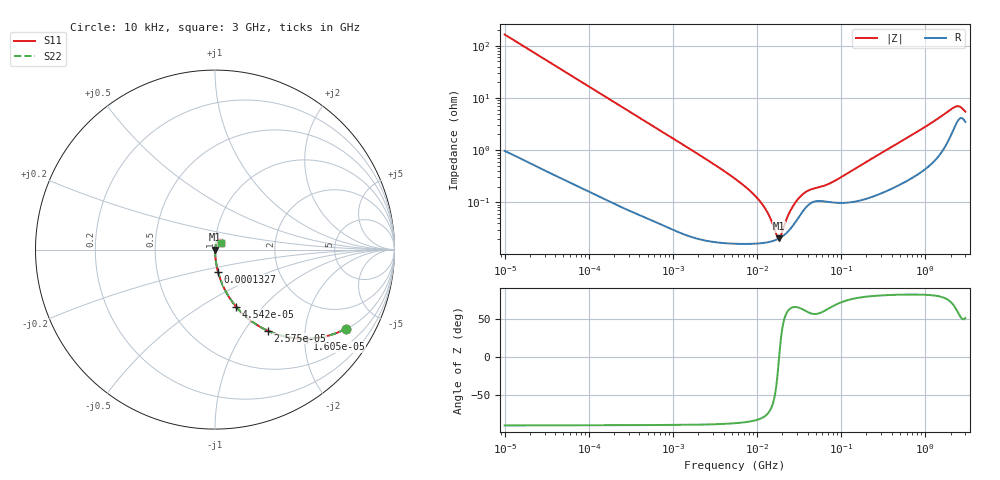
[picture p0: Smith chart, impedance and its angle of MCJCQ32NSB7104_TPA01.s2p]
! MCJCQ32NSB7104_TPA01  S-PARAMETER MODEL  ( Standard Model )
! Model Generated by TAIYO YUDEN Corporation (http://www.ty-top.com)
! Version 1.0
! TAIYO YUDEN Control No. 220601
! Copyright(c) 2015 TAIYO YUDEN CO.,LTD. All Rights Reserved.
! Product Description (link to TY-COMPAS)
! https://ds.yuden.co.jp/TYCOMPAS/or/detail?pn=MCJCQ32NSB7104KTPA01&u=M
! Products Name : Multilayer Ceramic Capacitors
! Characteristics :
!  Capacitance : 0.1 [uF] , Rated Voltage : 250 [V] , TCC : X7R
!  Case Size : 3.2 x 2.5 / 0.126 x 0.098 [mm/inch] , Thickness : 1.9 / 0.075 [mm/inch]
!  (Conditions: Temperature = 25 [degC] , DC Bias Voltage = 0 [V])
! External Node Assignments :
!  1  o---| |---o  2
! GND o---------o GND
! Frequency Range : 10kHz  -  3GHz  [ 401 STEP ]
# MHZ S RI R 50
! Freq[MHz].  S11 Real  S11 Imag  S21 Real  S21 Imag  S12 Real  S12 Imag  S22 Real  S22 Imag
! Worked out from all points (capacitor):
!   401 points, 10 kHz to 3 GHz, reference 50 ohm
!   read as one part in series: C = 96.7 nF near 10.65 kHz
!   lowest |Z| = 20.4 mohm at 18.15 MHz (marker M1)
!   series resonance near 18.34 MHz, so ESL is about 780 pH
!   S11 on the Smith chart (normalised r, x): 10 kHz: 1.02, -3.29; 16.05 kHz: 1.01, -2.05; 25.75 kHz: 1.01, -1.28; 45.42 kHz: 1.01, -0.73; 132.7 kHz: 1.00, -0.25; 3 GHz: 1.07, +0.08
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0.01  0.7287 -0.4417  0.2713 0.4417  0.2713 0.4417  0.7287 -0.4417
0.016047  0.513 -0.4966  0.487 0.4966  0.487 0.4966  0.513 -0.4966
0.02575  0.2925 -0.4514  0.7075 0.4514  0.7075 0.4514  0.2925 -0.4514
0.045421  0.1192 -0.3199  0.8808 0.3199  0.8808 0.3199  0.1192 -0.3199
0.082683  0.0404 -0.1923  0.9596 0.1923  0.9596 0.1923  0.0404 -0.1923
0.132681  0.0167 -0.1232  0.9833 0.1232  0.9833 0.1232  0.0167 -0.1232
0.683653  0.000997 -0.0246  0.999 0.0246  0.999 0.0246  0.000997 -0.0246
5.477226  0.000169 -0.00284  0.9998 0.00284  0.9998 0.00284  0.000169 -0.00284
11.31085  0.000166 -0.00095  0.9998 0.00095  0.9998 0.00095  0.000166 -0.00095
13.66633  0.000173 -0.000569  0.9998 0.000569  0.9998 0.000569  0.000173 -0.000569
17.04125  0.000193 -0.000142  0.9998 0.000142  0.9998 0.000142  0.000193 -0.000142
18.15044  0.000203 -1.98e-05  0.9998 1.98e-05  0.9998 1.98e-05  0.000203 -1.98e-05
19.33182  0.000215 0.000103  0.9998 -0.000103  0.9998 -0.000103  0.000215 0.000103
23.35767  0.000277 0.000483  0.9997 -0.000483  0.9997 -0.000483  0.000277 0.000483
28.22191  0.000405 0.000874  0.9996 -0.000874  0.9996 -0.000874  0.000405 0.000874
35.19136  0.000681 0.00127  0.9993 -0.00127  0.9993 -0.00127  0.000681 0.00127
45.28751  0.001 0.0015  0.999 -0.0015  0.999 -0.0015  0.001 0.0015
82.4407  0.000995 0.00234  0.999 -0.00234  0.999 -0.00234  0.000995 0.00234
374.4521  0.00185 0.0107  0.9982 -0.0107  0.9982 -0.0107  0.00185 0.0107
2188.735  0.0284 0.0573  0.9716 -0.0573  0.9716 -0.0573  0.0284 0.0573
2482.93  0.0396 0.0537  0.9604 -0.0537  0.9604 -0.0537  0.0396 0.0537
3000  0.0351 0.0395  0.9649 -0.0395  0.9649 -0.0395  0.0351 0.0395
